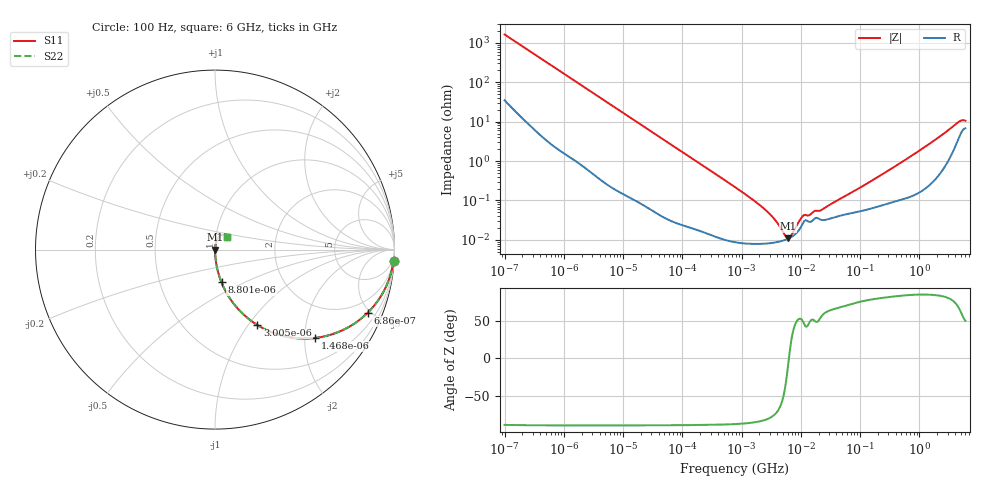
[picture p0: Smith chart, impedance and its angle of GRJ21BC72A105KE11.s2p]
!Murata Part Number: GRJ21BC72A105KE11
!These Parameters are Measured in Series Mode Connection
!Data Generated on Jun 19, 2026
!  o--ll--o
!Port1  Port2
!  o------o
!Operation Temp=25[degC], DC Bias Voltage=0[V]
!Freq. Start=100[Hz] Stop=6[GHz] 401[Steps]
# Hz S RI R 50
!Freq.(Hz) S11(Real) S11(Imag) S21(Real) S21(Imag) S12(Real) S12(Imag) S22(Real) S22(Imag)
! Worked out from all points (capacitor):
!   401 points, 100 Hz to 6 GHz, reference 50 ohm
!   read as one part in series: C = 973 nF near 109 Hz
!   lowest |Z| = 10.9 mohm at 6.075 MHz (marker M1)
!   series resonance near 6.291 MHz, so ESL is about 660 pH
!   S11 on the Smith chart (normalised r, x): 100 Hz: 2, -33; 686 Hz: 1.05, -4.81; 1.468 kHz: 1.02, -2.26; 3.005 kHz: 1.01, -1.11; 8.801 kHz: 1.00, -0.38; 6 GHz: 1.14, +0.16
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100  0.995 -0.0609  0.00504 0.0609  0.00504 0.0609  0.995 -0.0609
335  0.958 -0.1947  0.042 0.1947  0.042 0.1947  0.958 -0.1947
686  0.8502 -0.3521  0.1498 0.3521  0.1498 0.3521  0.8502 -0.3521
1468  0.5594 -0.4917  0.4406 0.4917  0.4406 0.4917  0.5594 -0.4917
2008  0.4065 -0.4865  0.5935 0.4865  0.5935 0.4865  0.4065 -0.4865
3005  0.2365 -0.4205  0.7635 0.4205  0.7635 0.4205  0.2365 -0.4205
4918  0.105 -0.3025  0.895 0.3025  0.895 0.3025  0.105 -0.3025
8801  0.0362 -0.1827  0.9638 0.1827  0.9638 0.1827  0.0362 -0.1827
40335  0.00217 -0.0417  0.9978 0.0417  0.9978 0.0417  0.00217 -0.0417
774597  9.21e-05 -0.00219  0.9999 0.00219  0.9999 0.00219  9.21e-05 -0.00219
2713602  8.14e-05 -0.000517  0.9999 0.000517  0.9999 0.000517  8.14e-05 -0.000517
3712478  8.63e-05 -0.000304  0.9999 0.000304  0.9999 0.000304  8.63e-05 -0.000304
5554849  0.000101 -6.92e-05  0.9999 6.92e-05  0.9999 6.92e-05  0.000101 -6.92e-05
6075234  0.000107 -1.94e-05  0.9999 1.94e-05  0.9999 1.94e-05  0.000107 -1.94e-05
6948629  0.000119 5.6e-05  0.9999 -5.6e-05  0.9999 -5.6e-05  0.000119 5.6e-05
1.039699e7  0.000234 0.000294  0.9998 -0.000294  0.9998 -0.000294  0.000234 0.000294
1.555665e7  0.000303 0.000383  0.9997 -0.000383  0.9997 -0.000383  0.000303 0.000383
2.327686e7  0.000318 0.000504  0.9997 -0.000504  0.9997 -0.000504  0.000318 0.000504
3.124326e8  0.000885 0.0059  0.9991 -0.0059  0.9991 -0.0059  0.000885 0.0059
1.431855e9  0.00301 0.0262  0.997 -0.0262  0.997 -0.0262  0.00301 0.0262
4.385646e9  0.0372 0.0819  0.9628 -0.0819  0.9628 -0.0819  0.0372 0.0819
6e9  0.0688 0.0707  0.9312 -0.0707  0.9312 -0.0707  0.0688 0.0707
